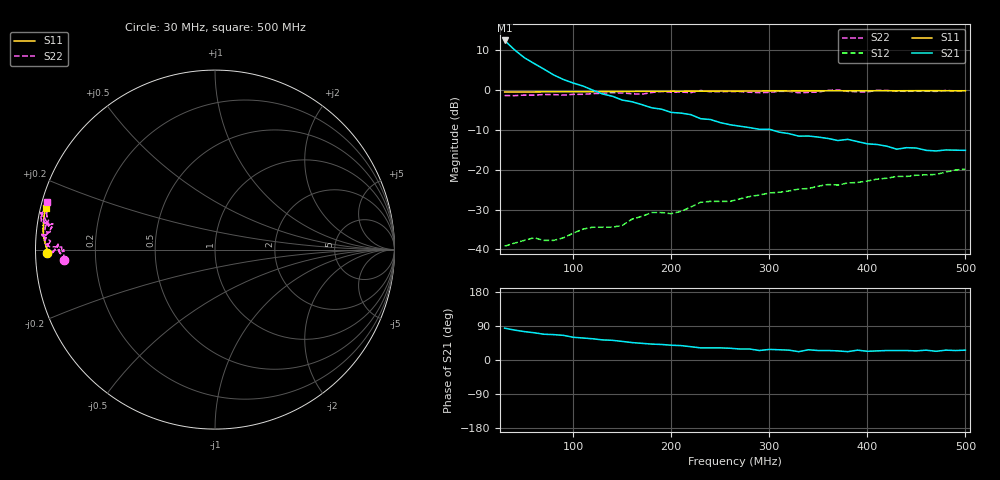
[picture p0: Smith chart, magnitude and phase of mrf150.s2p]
! Motorola RF High Power Semiconductors
! MRF150
! 50 V, 150 MHz 150 W N-Channel Linear RF Power MOSFET
! Vds = 50 V Id = 2 A
! Common Source S-Parameters: September 1998
# MHz S MA R 50
! f S11 S21 S12 S22
! MHz Mag Angle Mag Angle Mag Angle Mag Angle
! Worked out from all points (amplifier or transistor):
!   48 points, 30 MHz to 500 MHz, reference 50 ohm
!   highest |S21| = 12.3 dB at 30 MHz (marker M1)
!   |S21| within 3 dB of that: start of sweep to 43.43 MHz
!   unconditionally stable (mu >= 1): 76.9 MHz to 96.26 MHz; 120.8 MHz to 135 MHz; 168.7 MHz to 170.6 MHz
!   at 110 MHz: K = 0.99, MSG = 17.9 dB, |S12| = -34.9 dB
!   at 270 MHz: K = 0.65, MSG = 9.1 dB, |S12| = -27.3 dB
!   at 500 MHz: K = 0.67, MSG = 2.4 dB, |S12| = -19.9 dB
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30  0.936 -179.0  4.13 84.0  0.011 22.0  0.844 -176.0
40  0.936 -179.0  3.16 79.0  0.012 23.0  0.842 -180.0
50  0.936 -180.0  2.52 75.0  0.013 29.0  0.855 -179.0
60  0.937 180.0  2.13 72.0  0.014 36.0  0.854 179.0
70  0.939 179.0  1.81 68.0  0.013 42.0  0.87 179.0
80  0.94 179.0  1.53 67.0  0.013 45.0  0.868 -179.0
100  0.942 179.0  1.21 60.0  0.016 46.0  0.874 180.0
110  0.942 179.0  1.11 58.0  0.018 52.0  0.875 178.0
130  0.946 178.0  0.883 53.0  0.019 67.0  0.902 -179.0
150  0.949 177.0  0.741 49.0  0.02 63.0  0.91 -179.0
170  0.952 177.0  0.65 44.0  0.026 68.0  0.878 179.0
190  0.954 176.0  0.57 41.0  0.029 75.0  0.949 178.0
220  0.957 175.0  0.487 35.0  0.034 70.0  0.918 177.0
230  0.96 175.0  0.433 32.0  0.039 71.0  0.977 175.0
270  0.96 174.0  0.349 29.0  0.043 74.0  0.947 175.0
350  0.965 172.0  0.255 25.0  0.062 75.0  0.934 171.0
370  0.967 171.0  0.231 24.0  0.064 73.0  0.993 168.0
380  0.967 171.0  0.239 22.0  0.068 74.0  0.952 172.0
400  0.968 170.0  0.21 23.0  0.072 76.0  0.936 172.0
410  0.968 170.0  0.206 24.0  0.076 73.0  0.984 168.0
430  0.969 169.0  0.18 25.0  0.082 72.0  0.959 168.0
500  0.969 166.0  0.174 26.0  0.101 71.0  0.972 164.0
